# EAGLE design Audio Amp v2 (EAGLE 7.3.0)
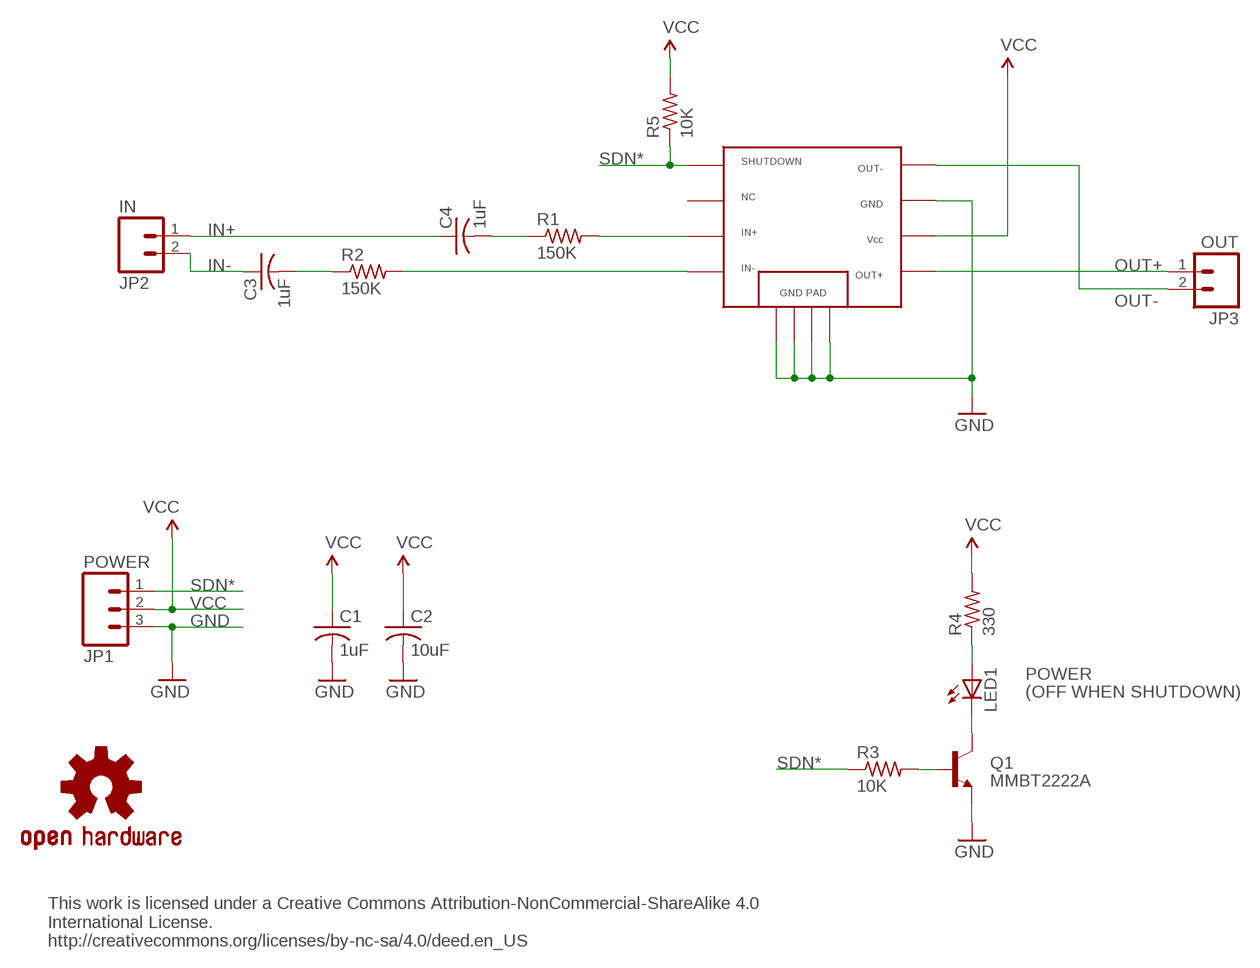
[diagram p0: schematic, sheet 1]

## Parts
C1  1uF  C-USC0805K  [C0805K]
C2  10uF  C-USC0805K  [C0805K]
C3  1uF  C-USC0805K  [C0805K]
C4  1uF  C-USC0805K  [C0805K]
JP1  POWER  M03PTH  [1X03]
JP2  IN  M02PTH  [1X02]
JP3  OUT  M02PTH  [1X02]
LED1  LED0603  [LED-0603]
Q1  MMBT2222A  TRANSISTOR_NPNSOT23-3  [SOT23-3]
R1  150K  R-US_M0805  [M0805]
R2  150K  R-US_M0805  [M0805]
R3  10K  R-US_M0805  [M0805]
R4  330  R-US_M0805  [M0805]
R5  10K  R-US_M0805  [M0805]
U1  TPA2005  [MSOP8]
U$2  OSHW-LOGOS  [OSHW-LOGO-S]

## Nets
GND: C1.2 C2.2 JP1.3 Q1.2(E) U1.7 U1.A U1.B U1.C U1.D
IN+: C4.1 JP2.1
IN+AMP: R1.2 U1.3
IN-: C3.1 JP2.2
IN-AMP: R2.2 U1.4
N$2: C4.2 R1.1
N$3: C3.2 R2.1
N$8: LED1.C Q1.3(C)
N$9: LED1.A R4.1
N$10: Q1.1(B) R3.2
OUT+: JP3.1 U1.5
OUT-: JP3.2 U1.8
SDN*: JP1.1 R3.1 R5.1 U1.1
VCC: C1.1 C2.1 JP1.2 R4.2 R5.2 U1.6
Unconnected: U1.NC

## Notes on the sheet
- POWER
- (OFF WHEN SHUTDOWN)
- This work is licensed under a Creative Commons Attribution-NonCommercial-ShareAlike 4.0
  International License.
  http://creativecommons.org/licenses/by-nc-sa/4.0/deed.en_US

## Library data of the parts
C1-C4 = adafruit:C-US: CAPACITOR, American symbol
JP1 = SparkFun:M03: Header 3 Standard 3-pin 0.1" header. Use with straight break away headers (SKU : PRT-00116), right angle break away headers (PRT-00553), swiss pins (PRT-00743), machine pins (PRT-00117), and female headers (PRT-00115). Molex polarized connector foot print use with SKU : PRT-08232 with associated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
JP2 JP3 = SparkFun:M02: Header 2
LED1 = SparkFun:LED: LEDs
Q1 = SparkFun:TRANSISTOR_NPN: Transistor NPN BJT configuration in SOT23 package. MMBT2222 is the common NPN we use. Double check BCE configuration again layout.
R1-R5 = adafruit:R-US_: RESISTOR, American symbol
U1 = TPA2005:TPA2005
U$2 = SparkFun:OSHW-LOGO: Open Source Hardware Logo This logo indicates the piece of hardware it is found on incorporates a OSHW license and/or adheres to the definition of open source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

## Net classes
0 default: clearance 0.254 mm
1 VCC: width 0.254 mm, clearance 0.254 mm

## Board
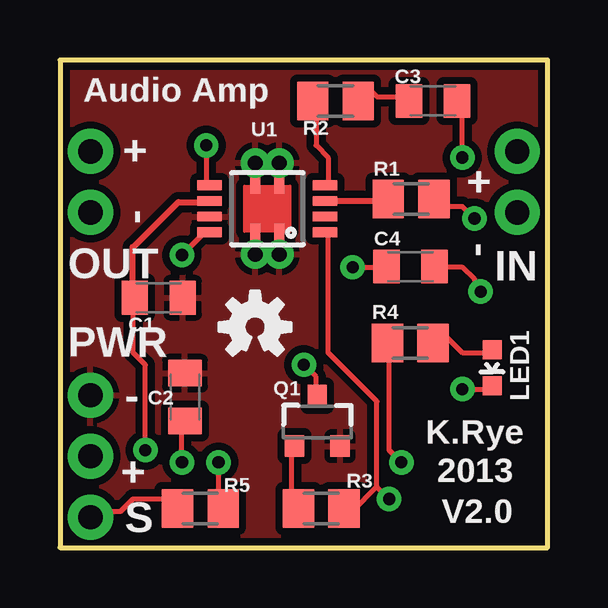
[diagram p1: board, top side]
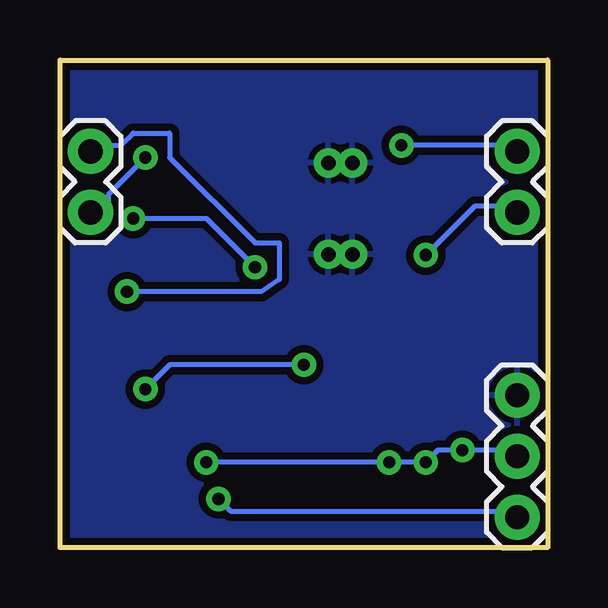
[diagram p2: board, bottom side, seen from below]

Size 20.32 x 20.32 mm. Coordinates in mm from the lower left corner, seen from the top.
Outline: 0,0 20.32,0 20.32,20.32 0,20.32 0,0
Copper layers (1*16): Top 0.035mm / dielectric 1.5mm / Bottom 0.035mm
Design rules "default": minimum track width 8mil, minimum drill 20mil, track to track 8mil, track to pad 8mil, pad to pad 8mil, via to via 8mil, smd to smd 8mil, copper to edge 8mil, drill to drill 8mil, minimum pad ring 12mil, minimum via ring 10mil, stop-mask expansion 4mil, vias tented up to drill 20mil, thermal gap 10mil

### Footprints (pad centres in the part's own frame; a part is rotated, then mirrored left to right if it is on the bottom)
C0805K = smd 1.1 x 1.4: 1 -1,0; 2 1,0
1X03 = drill 1.016 pad 1.88: 1 0,0; 2 2.54,0; 3 5.08,0
1X02 = drill 1.016 pad 1.88: 1 0,0; 2 2.54,0
LED-0603 = smd 0.8 x 0.8: A 0,-0.75; C 0,0.75
SOT23-3 = smd 0.8 x 0.9: 1 -0.95,-1; 2 0.95,-1; 3 0,1.1
M0805 = smd 1.3 x 1.6: 1 -0.95,0; 2 0.95,0
MSOP8 = smd 0.41 x 1.02: 1 -0.975,-2.4; 3 0.325,-2.4; 4 0.975,-2.4; 5 0.975,2.4; 6 0.325,2.4; 7 -0.325,2.4; 8 -0.975,2.4; NC -0.325,-2.4 | smd 1.02 x 0.41: 2 -1.13,0.5; 9 -1.13,-0.5; 10 1.13,-0.5; 11 1.13,0.5 | drill 0.61 pad 1.016: A -1.9,-0.5; B 1.91,-0.5; C 1.91,0.5; D -1.9,0.5

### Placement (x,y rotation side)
C1  4.11,10.41 0 top
C2  5.21,6.27 90 top
C3  15.54,18.62 180 top
C4  14.61,11.71 180 top
JP1  1.27,1.27 90 bottom
JP2  19.05,16.51 270 bottom
JP3  1.27,16.51 270 bottom
LED1  18.01,7.49 180 top
Q1  10.72,5.23 0 top
R1  14.63,14.53 180 top
R2  11.48,18.62 180 top
R3  10.88,1.63 180 top
R4  14.59,8.53 180 top
R5  5.85,1.63 0 top
U1  8.64,14.12 90 top
U$2  8.13,9.19 0 top

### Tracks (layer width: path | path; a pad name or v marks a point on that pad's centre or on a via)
GND
  pour Top (isolate 0.305): -0.94,21.95 21.72,21.95 21.59,-0.91 -1.12,-0.71
  pour Bottom (isolate 0.305): -0.94,21.92 21.62,22.02 21.59,-1.07 -1.24,-0.79
IN+  (via drill 0.51)
  Top 0.203: v17.53,10.67 17.27,11.18 16.76,11.68 15.75,11.68 C4.1
  Bottom 0.203: v17.53,10.67 11.94,10.67 11.18,11.18 11.18,12.7 12.19,12.7 15.75,16.26 15.75,17.27 17.27,17.27 17.78,16.76 18.8,16.76 JP2.1
IN+AMP
  Top 0.254: U1.3 13.68,14.45 R1.2
IN-  (via drill 0.51)
  Top 0.203: v16.76,16.26 16.76,18.29 C3.1
  Bottom 0.203: v16.76,16.26 18.29,14.73 18.29,14.22 18.8,14.22 JP2.2
IN-AMP
  Top 0.203: U1.4 11.18,15.24 11.18,16.26 10.67,16.76 10.67,18.29 R2.2
N$2  (via drill 0.51)
  Top 0.203: v12.19,11.68 13.21,11.68 C4.2 | v17.27,13.72 16.76,14.22 15.75,14.22 R1.1
  Bottom 0.203: v12.19,11.68 14.22,13.72 v17.27,13.72
N$3
  Top 0.203: C3.2 14.22,18.8 13.21,18.8 12.7,19.3 12.19,19.3 12.19,18.8 R2.1
N$8  (via drill 0.51)
  Top 0.203: v16.76,6.6 17.78,6.6 LED1.C | v10.16,7.62 10.67,7.11 10.67,6.6 Q1.3
  Bottom 0.203: v16.76,6.6 15.75,7.62 v10.16,7.62
N$9
  Top 0.203: LED1.A 17.78,8.13 16.76,8.13 15.75,9.14 R4.1
N$10
  Top 0.203: Q1.1 9.65,4.06 9.65,2.03 R3.2
OUT+  (via drill 0.51)
  Top 0.203: v6.1,16.76 6.1,15.24 U1.5
  Bottom 0.203: v6.1,16.76 1.52,16.76 JP3.1
OUT-  (via drill 0.51)
  Top 0.203: v5.08,12.19 6.1,13.21 U1.8
  Bottom 0.203: v5.08,12.19 3.05,14.22 1.52,14.22 JP3.2
SDN*  (via drill 0.51)
  Top 0.203: R5.1 4.57,2.03 3.05,2.03 2.54,1.52 1.52,1.52 JP1.1 | 13.21,2.54 13.21,6.1 11.18,8.13 11.18,13.21 U1.1 | 13.21,2.54 12.19,1.52 R3.1 | 13.21,2.54 v13.72,2.03
  Bottom 0.203: v13.72,2.03 13.21,1.52 1.52,1.52 JP1.1
VCC  (via drill 0.51)
  Top 0.203: v5.08,3.56 5.08,5.08 C2.1 | v3.56,4.06 3.56,7.62 3.05,8.13 3.05,10.16 C1.1 | v6.6,3.56 6.6,2.03 R5.2 | v14.22,3.56 13.72,4.06 13.72,8.64 R4.2
  Top 0.254: C1.1 3.02,10.41 3.02,12.52 3.05,12.52 4.93,14.4 6.19,14.4 U1.6
  Bottom 0.203: JP1.2 1.52,4.06 v3.56,4.06 4.57,4.06 v5.08,3.56 v6.6,3.56 v14.22,3.56

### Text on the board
Unrouted: This work is licensed under a Creative Commons Attribution-NonCommercial-ShareAlike 4.0 / International License. / http://creativecommons.org/licenses/by-nc-sa/4.0/deed.en_US
tPlace: + | + | - | - | OUT | IN | PWR | - | + | S
tNames: Audio Amp | K.Rye | 2013 | V2.0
